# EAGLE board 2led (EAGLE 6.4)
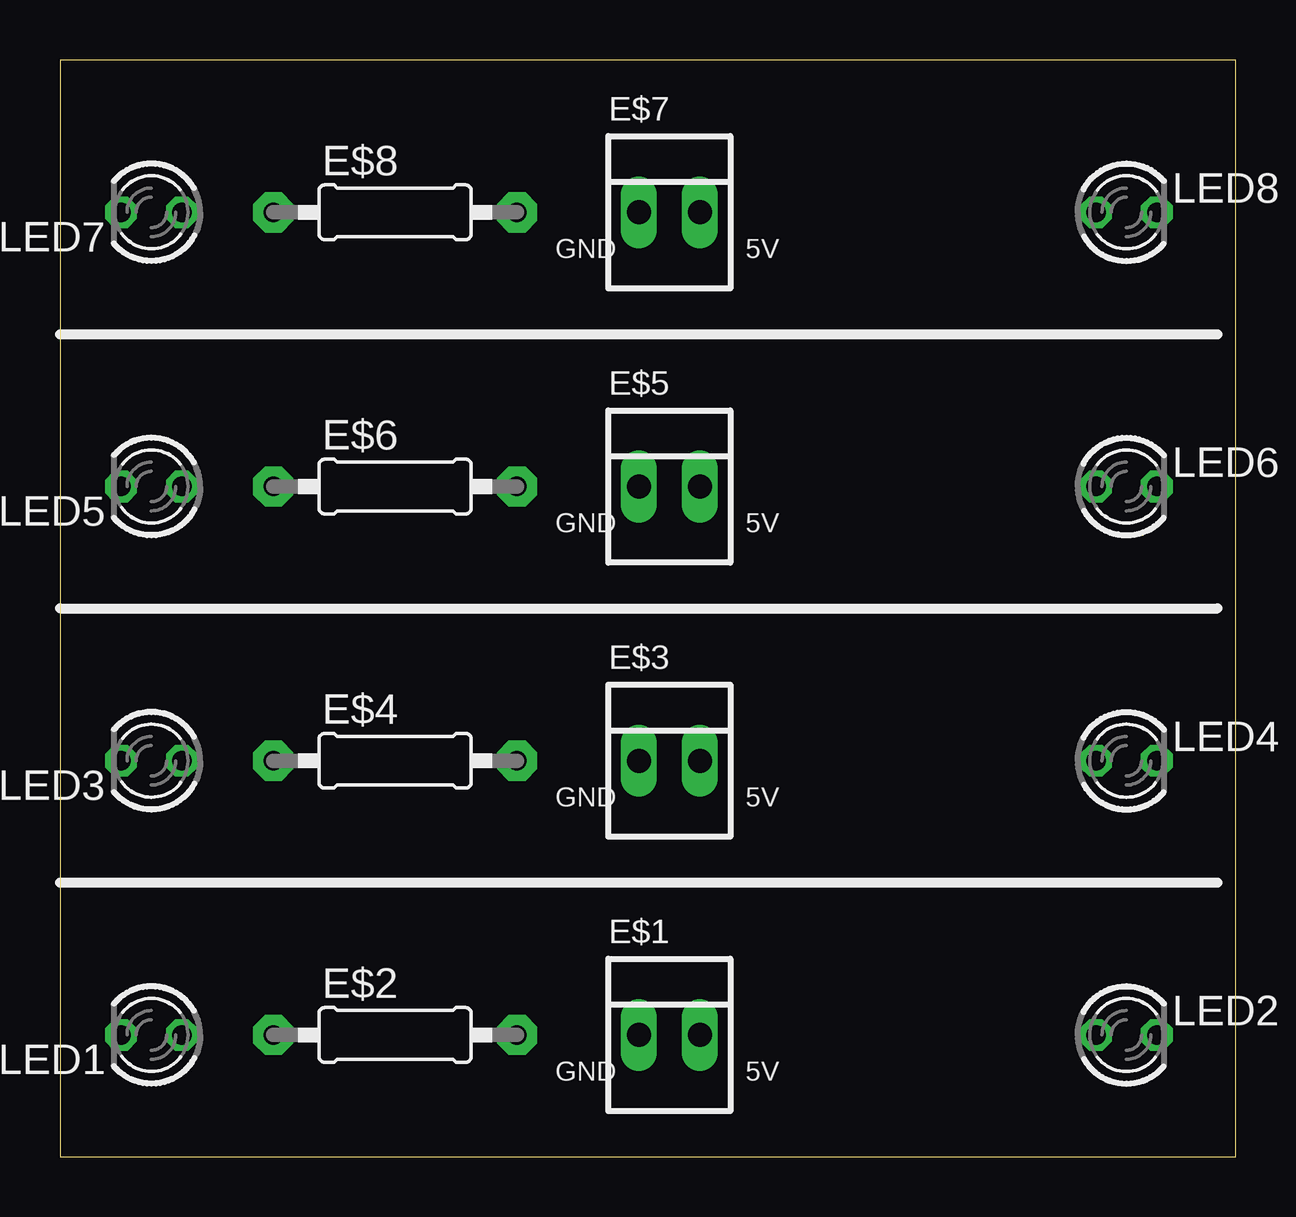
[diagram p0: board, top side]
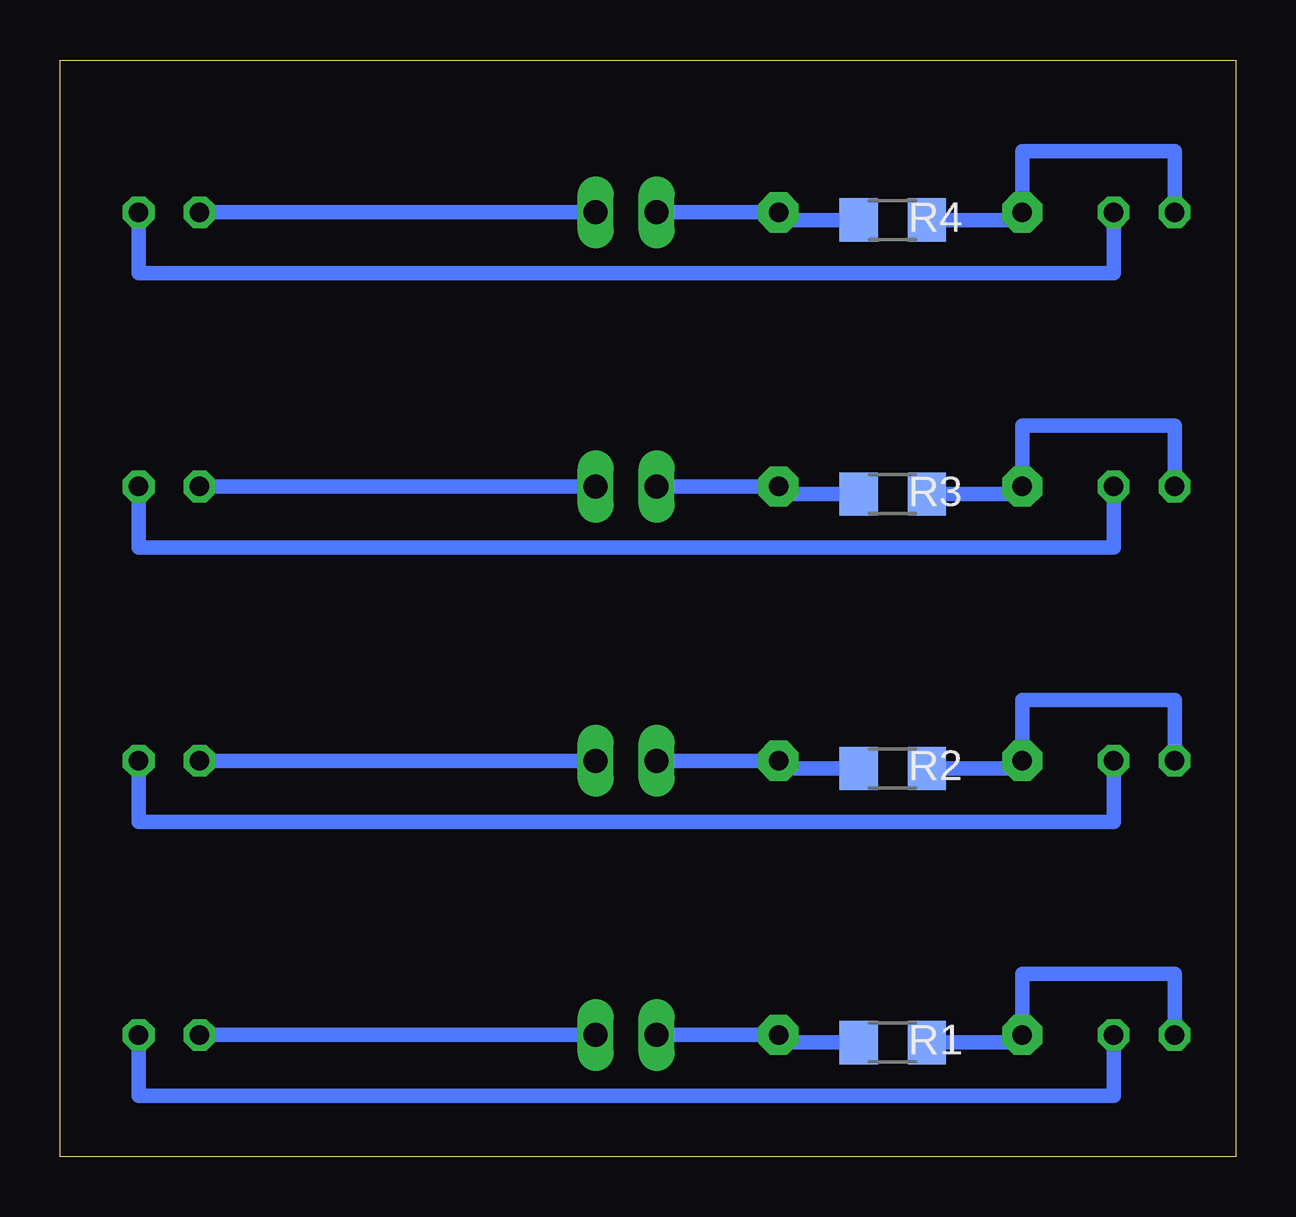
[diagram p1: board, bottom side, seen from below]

Size 49 x 45.72 mm. Coordinates in mm from the lower left corner, seen from the top.
Copper layers (1*16): Top 0.035mm / dielectric 1.5mm / Bottom 0.035mm
Design rules "default": minimum track width 10mil, minimum drill 24mil, track to track 8mil, track to pad 8mil, pad to pad 8mil, via to via 8mil, smd to smd 8mil, copper to edge 40mil, drill to drill 8mil, minimum pad ring 10mil, minimum via ring 8mil, stop-mask expansion 4mil, vias tented up to drill 0mil, thermal gap 10mil
Net classes: 0 default: width 0.457 mm; 1 power: width 0.914 mm

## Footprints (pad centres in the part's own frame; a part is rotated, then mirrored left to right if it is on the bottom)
22-23-2021 = drill 1 long: 1 -1.27,0; 2 1.27,0
0207/10 = drill 0.813 pad 1.676 octagon: 1 -5.08,0; 2 5.08,0
LED3MM = drill 0.813 octagon: A -1.27,0; K 1.27,0
R1206 = smd 1.6 x 1.803: 1 -1.422,0; 2 1.422,0

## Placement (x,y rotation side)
E$1  [22-23-2021]  25.4,5.08 0 top
E$2  [0207/10]  13.97,5.08 0 top
E$3  [22-23-2021]  25.4,16.51 0 top
E$4  [0207/10]  13.97,16.51 0 top
E$5  [22-23-2021]  25.4,27.94 0 top
E$6  [0207/10]  13.97,27.94 0 top
E$7  [22-23-2021]  25.4,39.37 0 top
E$8  [0207/10]  13.97,39.37 0 top
LED1  [LED3MM]  3.81,5.08 180 top
LED2  [LED3MM]  44.45,5.08 0 top
LED3  [LED3MM]  3.81,16.51 180 top
LED4  [LED3MM]  44.45,16.51 0 top
LED5  [LED3MM]  3.81,27.94 180 top
LED6  [LED3MM]  44.45,27.94 0 top
LED7  [LED3MM]  3.81,39.37 180 top
LED8  [LED3MM]  44.45,39.37 0 top
R1  1K  [R1206]  14.29,4.76 0 bottom
R2  1K  [R1206]  14.29,16.19 0 bottom
R3  1K  [R1206]  14.29,27.62 0 bottom
R4  1K  [R1206]  14.29,39.05 0 bottom

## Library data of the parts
E$1 E$3 E$5 E$7 = con-molex
E$2 E$4 E$6 E$8 = adafruit
LED1-LED8 = led
R1-R4 = smd-ipc

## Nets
S$1 [power]: E$1.1 E$2.2 R1.1
S$2 [power]: E$3.1 E$4.2 R2.1
S$3: LED1.A LED2.K
S$4: E$2.1 LED1.K R1.2
S$5 [power]: E$1.2 LED2.A
S$6 [power]: E$3.2 LED4.A
S$7: E$4.1 LED3.K R2.2
S$8: LED3.A LED4.K
S$9 [power]: E$5.1 E$6.2 R3.1
S$10 [power]: E$5.2 LED6.A
S$11: E$6.1 LED5.K R3.2
S$12: LED5.A LED6.K
S$13 [power]: E$7.1 E$8.2 R4.1
S$14 [power]: E$7.2 LED8.A
S$15: E$8.1 LED7.K R4.2
S$16: LED7.A LED8.K

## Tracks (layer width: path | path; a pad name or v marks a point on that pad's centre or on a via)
S$1
  Bottom 0.61: E$1.1 E$2.2 19.05,4.76 R1.1
S$2
  Bottom 0.61: E$3.1 E$4.2 19.05,16.19 R2.1
S$3
  Bottom 0.61: LED1.A 5.08,2.54 45.72,2.54 LED2.K
S$4
  Bottom 0.61: LED1.K 2.54,7.62 8.89,7.62 E$2.1 8.89,4.76 R1.2
S$5
  Bottom 0.61: LED2.A E$1.2
S$6
  Bottom 0.61: LED4.A E$3.2
S$7
  Bottom 0.61: LED3.K 2.54,19.05 8.89,19.05 E$4.1 8.89,16.19 R2.2
S$8
  Bottom 0.61: LED3.A 5.08,13.97 45.72,13.97 LED4.K
S$9
  Bottom 0.61: E$5.1 E$6.2 19.05,27.62 R3.1
S$10
  Bottom 0.61: LED6.A E$5.2
S$11
  Bottom 0.61: LED5.K 2.54,30.48 8.89,30.48 E$6.1 8.89,27.62 R3.2
S$12
  Bottom 0.61: LED5.A 5.08,25.4 45.72,25.4 LED6.K
S$13
  Bottom 0.61: E$7.1 E$8.2 19.05,39.05 R4.1
S$14
  Bottom 0.61: LED8.A E$7.2
S$15
  Bottom 0.61: LED7.K 2.54,41.91 8.89,41.91 E$8.1 8.89,39.05 R4.2
S$16
  Bottom 0.61: LED7.A 5.08,36.83 45.72,36.83 LED8.K

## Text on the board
tPlace: GND | 5V | GND | 5V | GND | 5V | GND | 5V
